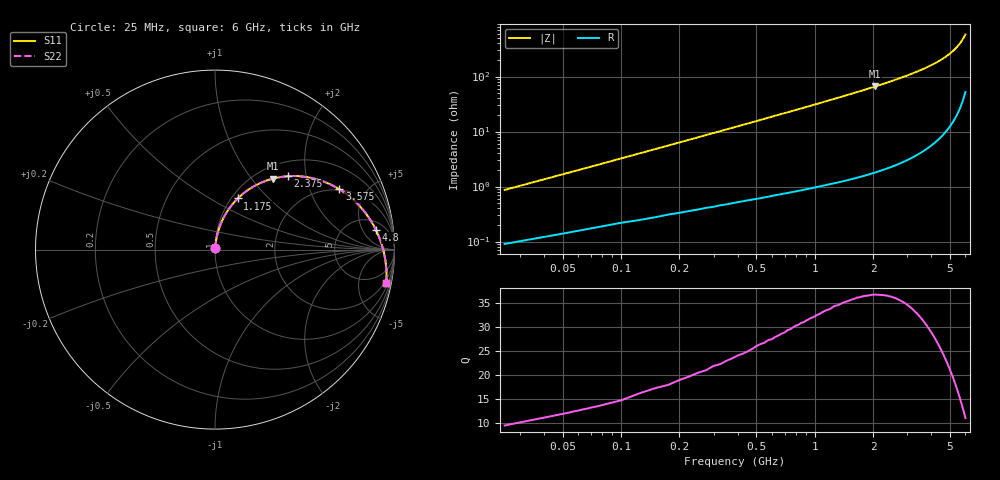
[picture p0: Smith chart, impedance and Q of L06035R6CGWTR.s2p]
!	AVX Thin Film Operation
!	Date:	March	2003
!	Description: Accu-L® Series Thin Film SMD RF Inductors
!	Part Number: L06035R6CGWTR
!	25MHz-6GHz
!	Serial	Measurements
#	mhz	S	db	R	50
!	S11	S11	S21	S21	S12	S12	S22	S22
!	dB	Phase	dB	Phase	dB	Phase	dB	Phase
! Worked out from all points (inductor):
!   240 points, 25 MHz to 6 GHz, reference 50 ohm
!   read as one part in series: L = 5.21 nH near 50 MHz
!   highest Q = 36.7 at 2.05 GHz (marker M1), where L = 5.12 nH
!   S11 on the Smith chart (normalised r, x): 25 MHz: 1.00, +0.02; 1.175 GHz: 1.07, +0.68; 2.375 GHz: 1.28, +1.57; 3.575 GHz: 1.96, +3.25; 4.8 GHz: 8, +10; 6 GHz: 1, -10
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25  -41.98 82.8  -0.01 -0.5  -0.01 -0.5  -41.98 82.8
50  -36.32 83.7  -0.01 -1.0  -0.01 -1.0  -36.32 83.7
75  -32.98 83.8  -0.02 -1.5  -0.02 -1.5  -32.98 83.8
100  -30.60 83.8  -0.02 -2.0  -0.02 -2.0  -30.60 83.8
175  -25.94 83.0  -0.04 -3.5  -0.04 -3.5  -25.94 83.0
275  -22.16 81.6  -0.06 -5.4  -0.06 -5.4  -22.16 81.6
400  -19.02 79.6  -0.10 -7.7  -0.10 -7.7  -19.02 79.6
575  -15.99 76.6  -0.17 -11.0  -0.17 -11.0  -15.99 76.6
775  -13.51 73.1  -0.27 -14.7  -0.27 -14.7  -13.51 73.1
1025  -11.22 68.7  -0.42 -19.3  -0.42 -19.3  -11.22 68.7
1175  -10.12 66.0  -0.53 -22.0  -0.53 -22.0  -10.12 66.0
1550  -7.93 59.4  -0.87 -28.7  -0.87 -28.7  -7.93 59.4
2025  -5.93 51.2  -1.42 -37.0  -1.42 -37.0  -5.93 51.2
2050  -5.84 50.8  -1.45 -37.4  -1.45 -37.4  -5.84 50.8
2375  -4.80 45.3  -1.90 -42.9  -1.90 -42.9  -4.80 45.3
3025  -3.23 34.6  -3.02 -53.5  -3.02 -53.5  -3.23 34.6
3575  -2.27 25.8  -4.19 -62.1  -4.19 -62.1  -2.27 25.8
4025  -1.65 18.8  -5.36 -69.0  -5.36 -69.0  -1.65 18.8
4800  -0.89 7.0  -7.98 -80.3  -7.98 -80.3  -0.89 7.0
5025  -0.72 3.6  -8.95 -83.5  -8.95 -83.5  -0.72 3.6
5575  -0.40 -4.7  -12.01 -90.9  -12.01 -90.9  -0.40 -4.7
6000  -0.24 -11.1  -15.56 -95.8  -15.56 -95.8  -0.24 -11.1
